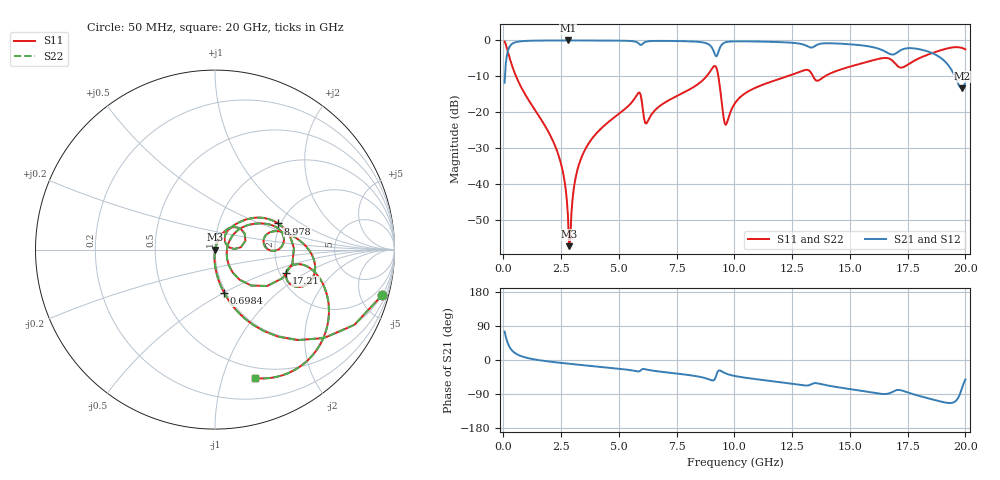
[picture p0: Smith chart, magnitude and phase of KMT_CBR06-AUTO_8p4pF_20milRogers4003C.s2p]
! Data measured by Modelithics Inc. support@modelithics.com 813-866-6335
! KEMET CBR06-AUTO 8.4pF, Pad Width= 0.851mm, Pad Length= 0.64mm, Pad Gap= 0.62mm, 20mil Rogers 4003C substrate Data, January 2022
# hz S ma R 50
! 2 Port Network Data from SP1.SP block
! freq  magS11  angS11  magS21  angS21  magS12  angS12  magS22  angS22
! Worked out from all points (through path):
!   401 points, 50 MHz to 20 GHz, reference 50 ohm
!   highest |S21| = -0.01 dB at 2.793 GHz (marker M1); lowest = -13.4 dB at 19.85 GHz (marker M2)
!   group delay of S21, straight-line fit = 16.1 ps
!   lowest |S11| = -57.4 dB at 2.843 GHz (marker M3), VSWR 1.00, Z = 50.1 - j0.115 ohm
!   |S11| at or under -10 dB: 544.6 MHz to 8.794 GHz (8.249 GHz wide, 177 % of centre); 9.303 GHz to 12.3 GHz (2.995 GHz wide, 27.7 % of centre); 13.4 GHz to 13.92 GHz (518.8 MHz wide, 3.8 % of centre)
!   |S22| runs from -57.4 to -0.3 dB; largest |S21 - S12| = 0
!   S11 on the Smith chart (normalised r, x): 50 MHz: 0.98, -7.44; 698.4 MHz: 0.98, -0.50; 8.978 GHz: 1.94, +0.66; 17.21 GHz: 2.17, -0.68; 20 GHz: 0.39, -1.29
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5e7  0.9664 -15.1  0.2569 74.9  0.2569 74.9  0.9664 -15.1
3.4925e8  0.4687 -63.2  0.8827 26.7  0.8827 26.7  0.4687 -63.2
6.98375e8  0.2461 -78.1  0.9686 11.8  0.9686 11.8  0.2461 -78.1
2.294375e9  0.0302 -94.8  0.9987 -6.3  0.9987 -6.3  0.0302 -94.8
2.593625e9  0.01356 -94.8  0.999 -8.4  0.999 -8.4  0.01356 -94.8
2.793125e9  0.003548 -85.3  0.999 -9.6  0.999 -9.6  0.003548 -85.3
2.843e9  0.001344 -58.8  0.999 -9.9  0.999 -9.9  0.001344 -58.8
3.391625e9  0.02388 74.4  0.9986 -13.3  0.9986 -13.3  0.02388 74.4
5.8355e9  0.1843 37.9  0.9166 -30.3  0.9166 -30.3  0.1843 37.9
6.184625e9  0.06925 33.1  0.9615 -25.0  0.9615 -25.0  0.06925 33.1
6.73325e9  0.1192 56.2  0.9856 -30.4  0.9856 -30.4  0.1192 56.2
8.977625e9  0.3814 22.5  0.8327 -52.9  0.8327 -52.9  0.3814 22.5
9.227e9  0.4101 -22.7  0.5988 -38.4  0.5988 -38.4  0.4101 -22.7
9.626e9  0.06639 -2.7  0.9432 -35.4  0.9432 -35.4  0.06639 -2.7
1.0025e10  0.1331 39.3  0.9716 -42.3  0.9716 -42.3  0.1331 39.3
1.336662e10  0.3335 -1.2  0.7976 -62.9  0.7976 -62.9  0.3335 -1.2
1.506238e10  0.4361 10.3  0.8807 -77.2  0.8807 -77.2  0.4361 10.3
1.670825e10  0.5563 -19.3  0.6518 -87.9  0.6518 -87.9  0.5563 -19.3
1.7207e10  0.4174 -18.1  0.732 -79.9  0.732 -79.9  0.4174 -18.1
1.895262e10  0.7321 -30.0  0.5647 -110.0  0.5647 -110.0  0.7321 -30.0
1.985038e10  0.7871 -64.4  0.2149 -74.7  0.2149 -74.7  0.7871 -64.4
2e10  0.7503 -72.5  0.2624 -51.2  0.2624 -51.2  0.7503 -72.5
